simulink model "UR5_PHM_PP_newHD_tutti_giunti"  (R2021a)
settings: Solver=ode14x  StartTime=0.0  StopTime=Sim.time  FixedStep=Sim.dt  MaxStep=Sim.dt  RelTol=1e-3  EnableMultiTasking=on
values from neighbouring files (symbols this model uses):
  alpha_n = 0.98*pi/180    (= 0.0171042266695)    [parameters.m]
  alpha_t = 30*pi/180    (= 0.523598775598)    [parameters.m]
  alpha_TTS = 0    [parameters.m]
  alpha_Tw_L = -6.9e-4    (= -0.00069)    [parameters.m]
  alpha_Tw_R = 3.9e-3    (= 0.0039)    [parameters.m]
  Beta_TTS = 0    [parameters.m]
  c1 = 1e-2    (= 0.01)    [parameters.m]
  c2 = 1e-2    (= 0.01)    [parameters.m]
  c3 = 1e-2    (= 0.01)    [parameters.m]
  c4 = 1e-2    (= 0.01)    [parameters.m]
  c5 = 1e-2    (= 0.01)    [parameters.m]
  c6 = 1e-2    (= 0.01)    [parameters.m]
  Cb1 = 1.8e3    (= 1800)    [parameters.m]
  Cb2 = 1.8e3    (= 1800)    [parameters.m]
  Cb3 = 1.8e3    (= 1800)    [parameters.m]
  Cb4 = 1.8e3    (= 1800)    [parameters.m]
  Cb5 = 1.8e3    (= 1800)    [parameters.m]
  Cb6 = 1.8e3    (= 1800)    [parameters.m]
  Cth_housing = 153.90    (= 153.9)    [parameters.m]
  Cth_w = 74.20    (= 74.2)    [parameters.m]
  dt_PP = 0.05    [parameters.m]
  Fric1 = [fc_1/2 1e1 fc_1 fv_1]    [parameters.m]
  Fric2 = [fc_2/2 1e1 fc_2 fv_2]    [parameters.m]
  Fric3 = [fc_3/2 1e1 fc_3 fv_3]    [parameters.m]
  Fric4 = [fc_4/2 1e1 fc_4 fv_4]    [parameters.m]
  Fric5 = [fc_5/2 1e1 fc_5 fv_5]    [parameters.m]
  Fric6 = [fc_6/2 1e1 fc_6 fv_6]    [parameters.m]
  Hth_housing = 0.30    (= 0.3)    [parameters.m]
  Hth_w = 1.14    [parameters.m]
  I_actual = I_actual(1:10,:)    [trajcutting.m]
  J_CS1 = 7.12e-5    (= 7.12e-05)    [parameters.m]
  J_CS2 = 7.12e-5    (= 7.12e-05)    [parameters.m]
  J_CS3 = 7.12e-5    (= 7.12e-05)    [parameters.m]
  J_CS4 = 6e-6    (= 6e-06)    [parameters.m]
  J_CS5 = 6e-6    (= 6e-06)    [parameters.m]
  J_CS6 = 6e-6    (= 6e-06)    [parameters.m]
  J_FS1 = 1.62e-7    (= 1.62e-07)    [parameters.m]
  J_FS2 = 1.62e-7    (= 1.62e-07)    [parameters.m]
  J_FS3 = 1.62e-7    (= 1.62e-07)    [parameters.m]
  J_FS4 = 4.97e-8    (= 4.97e-08)    [parameters.m]
  J_FS5 = 4.97e-8    (= 4.97e-08)    [parameters.m]
  J_FS6 = 4.97e-8    (= 4.97e-08)    [parameters.m]
  J_WG1 = 3.56e-5    (= 3.56e-05)    [parameters.m]
  J_WG2 = 3.56e-5    (= 3.56e-05)    [parameters.m]
  J_WG3 = 3.56e-5    (= 3.56e-05)    [parameters.m]
  J_WG4 = 3e-6    (= 3e-06)    [parameters.m]
  J_WG5 = 3e-6    (= 3e-06)    [parameters.m]
  J_WG6 = 3e-6    (= 3e-06)    [parameters.m]
  K_i = 1    [parameters.m]
  K_p = 1    [parameters.m]
  K_torsCS1 = 4.78e6    (= 4780000)    [parameters.m]
  K_torsCS2 = 4.78e6    (= 4780000)    [parameters.m]
  K_torsCS3 = 4.78e6    (= 4780000)    [parameters.m]
  K_torsCS4 = 1.06e6    (= 1060000)    [parameters.m]
  K_torsCS5 = 1.06e6    (= 1060000)    [parameters.m]
  K_torsCS6 = 1.06e6    (= 1060000)    [parameters.m]
  K_torsWG1 = 9.56e5    (= 956000)    [parameters.m]
  K_torsWG2 = 9.56e5    (= 956000)    [parameters.m]
  K_torsWG3 = 9.56e5    (= 956000)    [parameters.m]
  K_torsWG4 = 1.84e5    (= 184000)    [parameters.m]
  K_torsWG5 = 1.84e5    (= 184000)    [parameters.m]
  K_torsWG6 = 1.84e5    (= 184000)    [parameters.m]
  K_v = 1    [parameters.m]
  Kb1 = 0.51e8    (= 51000000)    [parameters.m]
  Kb2 = 0.51e8    (= 51000000)    [parameters.m]
  Kb3 = 0.51e8    (= 51000000)    [parameters.m]
  Kb4 = 1.98e7    (= 19800000)    [parameters.m]
  Kb5 = 1.98e7    (= 19800000)    [parameters.m]
  Kb6 = 1.98e7    (= 19800000)    [parameters.m]
  Km1 = 1.2e9    (= 1200000000)    [parameters.m]
  Km2 = 1.2e9    (= 1200000000)    [parameters.m]
  Km3 = 1.2e9    (= 1200000000)    [parameters.m]
  Km4 = 5.55e8    (= 555000000)    [parameters.m]
  Km5 = 5.55e8    (= 555000000)    [parameters.m]
  Km6 = 5.55e8    (= 555000000)    [parameters.m]
  Kt1 = 0.96e5    (= 96000)    [parameters.m]
  Kt2 = 0.96e5    (= 96000)    [parameters.m]
  Kt3 = 0.96e5    (= 96000)    [parameters.m]
  Kt4 = 1.15e4    (= 11500)    [parameters.m]
  Kt5 = 1.15e4    (= 11500)    [parameters.m]
  Kt6 = 1.15e4    (= 11500)    [parameters.m]
  L = Motor.L_2/2    [parameters.m]
  m2 = polyfit(Temp(:,2),pBn_UR5_f_Temp(:,2),1)    [parameters.m]
  mb2 = polyfit(Temp(:,8),pBn_UR5_f_Temp(:,8),1)    [parameters.m]
  pickTime = t_pick(traj)    [parameters.m]
  placeTime = t_place(traj)    [parameters.m]
  q0 = q_target(1,:)    [testlaw_PP.m]
  q_CS01 = x(6)    [parameters.m]
  q_CS02 = x(6)    [parameters.m]
  q_CS03 = x(6)    [parameters.m]
  q_CS04 = x(6)    [parameters.m]
  q_CS05 = x(6)    [parameters.m]
  q_CS06 = x(6)    [parameters.m]
  q_WG01 = x(1)    [parameters.m]
  q_WG02 = x(1)    [parameters.m]
  q_WG03 = x(1)    [parameters.m]
  q_WG04 = x(1)    [parameters.m]
  q_WG05 = x(1)    [parameters.m]
  q_WG06 = x(1)    [parameters.m]
  quant_i = [Motor.imax1 Motor.imax2      Motor.imax3 Motor.imax4 Motor.imax5 Motor.imax6]/2^16    [parameters.m]
  R = Motor.R_2/2    [parameters.m]
  rg1 = 0.028    [parameters.m]
  rg2 = 0.028    [parameters.m]
  rg3 = 0.028    [parameters.m]
  rg4 = 0.0155    [parameters.m]
  rg5 = 0.0155    [parameters.m]
  rg6 = 0.0155    [parameters.m]
  sigma_p = 444.29    [parameters.m]
  sigma_v = 2*pi*1000    (= 6283.18530718)    [parameters.m]
  stiff_red = 1    [parameters.m]
  T_0 = Sim.temp    [parameters.m]
  T_switch = 1e-4    (= 0.0001)    [parameters.m]
  tau_i = 1/(fc_i*2*pi)    (= 7.95774715459e-05)    [parameters.m]
  U_s = 48    [parameters.m]
  var_i = 1e-1*[.0167 .0184 .0144 .0016      .0011 .0007]    [parameters.m]
  var_p = 1e-6*[.0943 .3877      .3478 .5436 .3400 .2081]    [parameters.m]
  var_v = 1e-4*[.0738 .1452      .1564 .4623 .1824 .0917]    [parameters.m]
  Wf_TTS_0 = 0    [parameters.m]
  Wf_TTS_ONOFF = 0    [parameters.m]
  x2_01 = x(3)    [parameters.m]
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undefined symbols (not defined in the file or in its folder): deg, Driver1, Driver2, Driver3, Driver4, Driver5, Driver6, elseif, geom, Ground, J1, J2, J3, J4, J5, J6, kg, L1, L2, L3, L4, L5, L6, LINK0, LINK1, LINK2, LINK3, LINK4, LINK5, LINK6, m, Motor, N, payload, ROBOTIQ_FT, s, Sim, Tool, X, Y, Z
libraries: sm_lib x35, nesl_utility x30, simulink x23, simulink_extras x11, spsTriangleGeneratorLib x6
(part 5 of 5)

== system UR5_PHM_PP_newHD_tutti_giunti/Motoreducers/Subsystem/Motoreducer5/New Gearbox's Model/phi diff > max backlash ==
  In2 : Inport
  In3 : Inport  Port=2
  Action Port : ActionPort  PropagateVarSize=During execution  ActionPortLabel=elseif(u2>u3)
  Add1 : Sum  Inputs=+|-
  Add2 : Sum  Inputs=+|+
  Add4 : Sum  Inputs=+|+
  Compare To Zero : simulink/Logic and Bit Operations/Compare To Zero  relop=<=  OutDataTypeStr=uint8
  Constant : Constant  Value=0
  Constant3 : Constant  Value=J5.clearance
  Cs_shaft [Nm/(rad/s)] : Gain  Gain=J5.C
  Ks_shaft [Nm/rad] : Gain  Gain=J5.K
  MinMax : MinMax  Inputs=2
  Switch : Switch  Criteria=u2 > Threshold
  Out1 : Outport  VectorParamsAs1DForOutWhenUnconnected=off
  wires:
  Switch/1 -> Out1/1
  Add2/1 -> Switch/3
  MinMax/1 -> Add2/2
  Add4/1 -> Compare To Zero/1
  Constant/1 -> Switch/1
  Compare To Zero/1 -> Switch/2
  Add1/1 -> Ks_shaft [Nm/rad]/1
  Constant3/1 -> Add1/2
  In2/1 -> Add1/1
  In3/1 -> Cs_shaft [Nm/(rad/s)]/1
  Cs_shaft [Nm/(rad/s)]/1 -> MinMax/2, Add4/2
  Ks_shaft [Nm/rad]/1 -> Add2/1, MinMax/1, Add4/1

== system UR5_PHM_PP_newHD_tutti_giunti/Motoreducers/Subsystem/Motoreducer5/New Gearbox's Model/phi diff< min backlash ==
  In2 : Inport
  In3 : Inport  Port=2
  Action Port : ActionPort  PropagateVarSize=During execution  ActionPortLabel=elseif( u2<u4)
  Add1 : Sum  Inputs=+|-
  Add2 : Sum  Inputs=+|+
  Add4 : Sum  Inputs=+|+
  Compare To Zero : simulink/Logic and Bit Operations/Compare To Zero  relop=>=  OutDataTypeStr=uint8
  Constant : Constant  Value=0
  Constant1 : Constant  Value=0
  Cs_shaft [Nm/(rad/s)] : Gain  Gain=J5.C
  Ks_shaft [Nm/rad] : Gain  Gain=J5.K
  MinMax : MinMax  Function=max  Inputs=2
  Switch : Switch  Criteria=u2 > Threshold
  Out1 : Outport  VectorParamsAs1DForOutWhenUnconnected=off
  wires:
  Switch/1 -> Out1/1
  Add2/1 -> Switch/3
  MinMax/1 -> Add2/2
  Add4/1 -> Compare To Zero/1
  Constant/1 -> Switch/1
  Compare To Zero/1 -> Switch/2
  Add1/1 -> Ks_shaft [Nm/rad]/1
  Constant1/1 -> Add1/2
  In2/1 -> Add1/1
  In3/1 -> Cs_shaft [Nm/(rad/s)]/1
  Cs_shaft [Nm/(rad/s)]/1 -> MinMax/2, Add4/2
  Ks_shaft [Nm/rad]/1 -> Add2/1, MinMax/1, Add4/1

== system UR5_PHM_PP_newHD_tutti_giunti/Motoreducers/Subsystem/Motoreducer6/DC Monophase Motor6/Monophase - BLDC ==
  Vset : Inport
  qdm : Inport  Port=2
  Phase A : Subsystem
  Torque constant [Nm/A] : Gain  Gain=Motor.kc_6
  T : Outport  VectorParamsAs1DForOutWhenUnconnected=off
  i : Outport  Port=2  VectorParamsAs1DForOutWhenUnconnected=off
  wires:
  Vset/1 -> Phase A/1(Vset)
  Torque constant [Nm/A]/1 -> T/1
  Phase A/1(i) -> Torque constant [Nm/A]/1, i/1
  qdm/1 -> Phase A/2(qdm)

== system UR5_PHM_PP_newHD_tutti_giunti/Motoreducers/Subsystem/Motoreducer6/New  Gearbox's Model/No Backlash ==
  qm : Inport
  q : Inport  Port=2
  qdm : Inport  Port=3
  qd : Inport  Port=4
  Action Port : ActionPort  PropagateVarSize=During execution  ActionPortLabel=if(u1<=1e-10)
  Circular spline : Subsystem
  Flexspline (rad) : Subsystem
  Flexspline (tang) : Subsystem
  Wave Generator : Subsystem
  Ccs->giunto : Outport
  Cwg->rotore : Outport  Port=2
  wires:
  Flexspline (tang)/1(y1) -> Flexspline (rad)/4(y1), Circular spline/1(y1)
  Flexspline (rad)/2(x2) -> Circular spline/3(x2), Flexspline (tang)/2(x2)
  q/1 -> Circular spline/4(q)
  qd/1 -> Circular spline/5(qd)
  Circular spline/1(C1) -> Ccs->giunto/1
  Circular spline/2(q_CS) -> Flexspline (rad)/3(q_CS)
  qm/1 -> Wave Generator/1(qm)
  qdm/1 -> Wave Generator/2(qdm)
  Flexspline (rad)/3(C_WG->FS) -> Wave Generator/3(C_FS->WG)
  Wave Generator/1(Cwg->rotore) -> Cwg->rotore/1
  Wave Generator/2(qm_WG) -> Flexspline (rad)/1(qm_WG)
  Wave Generator/3(qdm_WG) -> Flexspline (rad)/2(qdm_WG)
  Flexspline (rad)/1(y2) -> Circular spline/2(y2), Flexspline (tang)/1(y2)

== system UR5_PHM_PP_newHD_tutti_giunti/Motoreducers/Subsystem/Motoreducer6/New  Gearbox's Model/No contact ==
  In2 : Inport
  In3 : Inport  Port=2
  Action Port : ActionPort  PropagateVarSize=During execution  ActionPortLabel=else
  1/(2-1/eta_dir) : Gain  Gain=0
  Add4 : Sum  Inputs=+|+
  Out3 : Outport  VectorParamsAs1DForOutWhenUnconnected=off
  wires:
  Add4/1 -> 1/(2-1/eta_dir)/1
  In3/1 -> Add4/2
  In2/1 -> Add4/1
  1/(2-1/eta_dir)/1 -> Out3/1

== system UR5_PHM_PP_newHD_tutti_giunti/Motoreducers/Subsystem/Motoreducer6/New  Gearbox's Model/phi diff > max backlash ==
  In2 : Inport
  In3 : Inport  Port=2
  Action Port : ActionPort  PropagateVarSize=During execution  ActionPortLabel=elseif(u2>u3)
  Add1 : Sum  Inputs=+|-
  Add2 : Sum  Inputs=+|+
  Add4 : Sum  Inputs=+|+
  Compare To Zero : simulink/Logic and Bit Operations/Compare To Zero  relop=<=  OutDataTypeStr=uint8
  Constant : Constant  Value=0
  Constant3 : Constant  Value=J6.clearance
  Cs_shaft [Nm/(rad/s)] : Gain  Gain=J6.C
  Ks_shaft [Nm/rad] : Gain  Gain=J6.K
  MinMax : MinMax  Inputs=2
  Switch : Switch  Criteria=u2 > Threshold
  Out1 : Outport  VectorParamsAs1DForOutWhenUnconnected=off
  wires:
  Switch/1 -> Out1/1
  Add2/1 -> Switch/3
  MinMax/1 -> Add2/2
  Add4/1 -> Compare To Zero/1
  Constant/1 -> Switch/1
  Compare To Zero/1 -> Switch/2
  Add1/1 -> Ks_shaft [Nm/rad]/1
  Constant3/1 -> Add1/2
  In2/1 -> Add1/1
  In3/1 -> Cs_shaft [Nm/(rad/s)]/1
  Cs_shaft [Nm/(rad/s)]/1 -> MinMax/2, Add4/2
  Ks_shaft [Nm/rad]/1 -> Add2/1, MinMax/1, Add4/1

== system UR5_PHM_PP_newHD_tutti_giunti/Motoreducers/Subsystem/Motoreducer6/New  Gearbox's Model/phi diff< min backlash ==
  In2 : Inport
  In3 : Inport  Port=2
  Action Port : ActionPort  PropagateVarSize=During execution  ActionPortLabel=elseif( u2<u4)
  Add1 : Sum  Inputs=+|-
  Add2 : Sum  Inputs=+|+
  Add4 : Sum  Inputs=+|+
  Compare To Zero : simulink/Logic and Bit Operations/Compare To Zero  relop=>=  OutDataTypeStr=uint8
  Constant : Constant  Value=0
  Constant1 : Constant  Value=0
  Cs_shaft [Nm/(rad/s)] : Gain  Gain=J6.C
  Ks_shaft [Nm/rad] : Gain  Gain=J6.K
  MinMax : MinMax  Function=max  Inputs=2
  Switch : Switch  Criteria=u2 > Threshold
  Out1 : Outport  VectorParamsAs1DForOutWhenUnconnected=off
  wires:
  Switch/1 -> Out1/1
  Add2/1 -> Switch/3
  MinMax/1 -> Add2/2
  Add4/1 -> Compare To Zero/1
  Constant/1 -> Switch/1
  Compare To Zero/1 -> Switch/2
  Add1/1 -> Ks_shaft [Nm/rad]/1
  Constant1/1 -> Add1/2
  In2/1 -> Add1/1
  In3/1 -> Cs_shaft [Nm/(rad/s)]/1
  Cs_shaft [Nm/(rad/s)]/1 -> MinMax/2, Add4/2
  Ks_shaft [Nm/rad]/1 -> Add2/1, MinMax/1, Add4/1

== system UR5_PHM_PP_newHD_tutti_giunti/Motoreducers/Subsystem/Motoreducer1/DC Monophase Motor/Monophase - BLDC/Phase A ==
  Vset : Inport
  qdm : Inport  Port=2
  Add : Sum  Inputs=-+
  Gain : Gain  Gain=Motor.kv_1
  Saturation : Saturate  UpperLimit=Motor.imax1  LowerLimit=-Motor.imax1
  Transfer Fcn : TransferFcn  Numerator=[1/Motor.R_123]  Denominator=[Motor.L_123/Motor.R_123 1]
  i : Outport  VectorParamsAs1DForOutWhenUnconnected=off
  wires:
  Gain/1 -> Add/1
  Transfer Fcn/1 -> Saturation/1
  qdm/1 -> Gain/1
  Add/1 -> Transfer Fcn/1
  Vset/1 -> Add/2
  Saturation/1 -> i/1

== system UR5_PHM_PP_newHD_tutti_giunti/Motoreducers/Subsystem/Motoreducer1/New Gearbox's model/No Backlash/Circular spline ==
  y2 : Inport
  x2 : Inport  Port=2
  y1 : Inport  Port=3
  q : Inport  Port=4
  qd : Inport  Port=5
  1/J_CS : Gain  Gain=1/J_CS1
  Add : Sum  Inputs=+--
  Add1 : Sum  Inputs=+-
  Add2 : Sum  Inputs=+-
  Add3 : Sum
  Add4 : Sum  Inputs=-+-
  Integrator : Integrator
  Integrator1 : Integrator  InitialCondition=q_CS01
  K_torsCS : Gain  Gain=K_torsCS1
  c : Gain  Gain=c1
  cos(alpha_t) : Gain  Gain=cos(alpha_t)
  cos(alpha_t)2 : Gain  Gain=cos(alpha_t)
  rg*Km*cos(alpha_t) : Gain  Gain=rg1*Km1*cos(alpha_t)
  sin(alpha_t) : Gain  Gain=sin(alpha_t)
  C1 : Outport
  q_CS : Outport  Port=2
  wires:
  cos(alpha_t)/1 -> Add4/3
  Add4/1 -> rg*Km*cos(alpha_t)/1
  x2/1 -> sin(alpha_t)/1
  y1/1 -> cos(alpha_t)/1
  sin(alpha_t)/1 -> Add4/2
  cos(alpha_t)2/1 -> Add4/1
  y2/1 -> cos(alpha_t)2/1
  Integrator/1 -> Add2/1, Integrator1/1
  Add3/1 -> C1/1
  1/J_CS/1 -> Integrator/1
  Add1/1 -> K_torsCS/1
  Add/1 -> 1/J_CS/1
  Integrator1/1 -> q_CS/1, Add1/1
  c/1 -> Add3/2, Add/3
  K_torsCS/1 -> Add3/1, Add/2
  Add2/1 -> c/1
  rg*Km*cos(alpha_t)/1 -> Add/1
  qd/1 -> Add2/2
  q/1 -> Add1/2

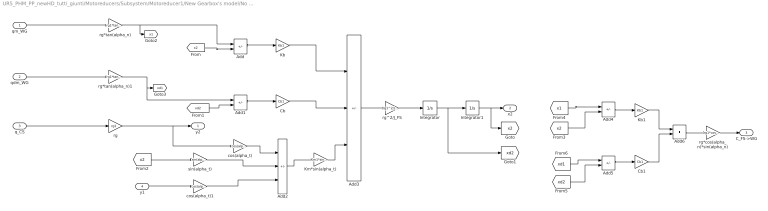
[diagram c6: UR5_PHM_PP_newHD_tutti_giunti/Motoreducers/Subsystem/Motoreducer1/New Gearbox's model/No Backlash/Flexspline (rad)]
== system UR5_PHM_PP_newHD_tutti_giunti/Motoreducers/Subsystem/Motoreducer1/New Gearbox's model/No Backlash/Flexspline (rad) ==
  qm_WG : Inport
  qdm_WG : Inport  Port=2
  q_CS : Inport  Port=3
  y1 : Inport  Port=4
  Add{,1,4..5} (4 alike) : Sum  Inputs=+-
  Add2 : Sum  Inputs=-+-
  Add3 : Sum  Inputs=++-
  Add6 : Sum
  Cb : Gain  Gain=Cb1
  Cb1 : Gain  Gain=Cb1
  Integrator : Integrator
  Integrator1 : Integrator  InitialCondition=x2_01
  Kb : Gain  Gain=Kb1
  Kb1 : Gain  Gain=Kb1
  Km*sin(alpha_t) : Gain  Gain=Km1*sin(alpha_t)
  cos(alpha_t) : Gain  Gain=cos(alpha_t)
  cos(alpha_t)1 : Gain  Gain=cos(alpha_t)
  rg : Gain  Gain=rg1
  rg*cos(alpha_n)*sin(alpha_n) : Gain  Gain=rg1*cos(alpha_n)*sin(alpha_n)
  rg*tan(alpha_n) : Gain  Gain=rg1*tan(alpha_n)
  rg*tan(alpha_n)1 : Gain  Gain=rg1*tan(alpha_n)
  rg^2/J_FS : Gain  Gain=rg1^2/J_FS1
  sin(alpha_t) : Gain  Gain=sin(alpha_t)
  y2 : Outport
  x2 : Outport  Port=2
  C_FS->WG : Outport  Port=3
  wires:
  Cb1/1 -> Add6/2
  Kb1/1 -> Add6/1
  sin(alpha_t)/1 -> Add2/2
  Add4/1 -> Kb1/1
  cos(alpha_t)1/1 -> Add2/3
  Add2/1 -> Km*sin(alpha_t)/1
  y1/1 -> cos(alpha_t)1/1
  Cb/1 -> Add3/2
  qdm_WG/1 -> rg*tan(alpha_n)1/1
  q_CS/1 -> rg/1
  Kb/1 -> Add3/1
  Km*sin(alpha_t)/1 -> Add3/3
  Add1/1 -> Cb/1
  rg/1 -> cos(alpha_t)/1, y2/1
  Integrator1/1 -> [x2], x2/1
  Add3/1 -> rg^2/J_FS/1
  rg^2/J_FS/1 -> Integrator/1
  cos(alpha_t)/1 -> Add2/1
  Add/1 -> Kb/1
  Integrator/1 -> [xd2], Integrator1/1
  Add5/1 -> Cb1/1
  [x2] -> sin(alpha_t)/1
  rg*tan(alpha_n)1/1 -> [xd1], Add1/1
  Add6/1 -> rg*cos(alpha_n)*sin(alpha_n)/1
  rg*cos(alpha_n)*sin(alpha_n)/1 -> C_FS->WG/1
  qm_WG/1 -> rg*tan(alpha_n)/1
  [xd2] -> Add1/2
  [x2] -> Add/2
  rg*tan(alpha_n)/1 -> [x1], Add/1
  [x2] -> Add4/2
  [x1] -> Add4/1
  [xd2] -> Add5/2
  [xd1] -> Add5/1

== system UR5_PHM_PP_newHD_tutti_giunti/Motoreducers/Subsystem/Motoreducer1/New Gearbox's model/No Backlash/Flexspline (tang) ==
  y2 : Inport
  x2 : Inport  Port=2
  Add : Sum  Inputs=+-
  Add4 : Sum  Inputs=-+-
  Integrator : Integrator
  Integrator1 : Integrator  InitialCondition=y1_01
  Km*cos(alpha_t) : Gain  Gain=Km1*cos(alpha_t)
  Kt/rg^2 : Gain  Gain=Kt1/rg1^2
  cos(alpha_t) : Gain  Gain=cos(alpha_t)
  cos(alpha_t)2 : Gain  Gain=cos(alpha_t)
  rg^2/J_FS : Gain  Gain=rg1^2/J_FS1
  sin(alpha_t) : Gain  Gain=sin(alpha_t)
  y1 : Outport
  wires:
  Integrator/1 -> Integrator1/1
  y2/1 -> cos(alpha_t)2/1
  Integrator1/1 -> cos(alpha_t)/1, Kt/rg^2/1, y1/1
  Add4/1 -> Km*cos(alpha_t)/1
  Kt/rg^2/1 -> Add/2
  rg^2/J_FS/1 -> Integrator/1
  Add/1 -> rg^2/J_FS/1
  x2/1 -> sin(alpha_t)/1
  Km*cos(alpha_t)/1 -> Add/1
  sin(alpha_t)/1 -> Add4/2
  cos(alpha_t)2/1 -> Add4/1
  cos(alpha_t)/1 -> Add4/3

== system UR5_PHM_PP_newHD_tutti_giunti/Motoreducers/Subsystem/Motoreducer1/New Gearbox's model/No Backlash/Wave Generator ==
  qm : Inport
  qdm : Inport  Port=2
  C_FS->WG : Inport  Port=3
  1/J_WG : Gain  Gain=1/J_WG1
  Add : Sum  Inputs=+-
  Add1 : Sum  Inputs=+-
  Add2 : Sum
  Add4 : Sum  Inputs=+-
  Integrator1 : Integrator
  Integrator2 : Integrator  InitialCondition=q_WG01
  K_torsWG : Gain  Gain=K_torsWG1
  c : Gain  Gain=c1
  Cwg->rotore : Outport
  qm_WG : Outport  Port=2
  qdm_WG : Outport  Port=3
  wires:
  Integrator1/1 -> qdm_WG/1, Add1/2, Integrator2/1
  Add1/1 -> c/1
  Integrator2/1 -> qm_WG/1, Add/2
  Add2/1 -> Cwg->rotore/1, Add4/1
  1/J_WG/1 -> Integrator1/1
  c/1 -> Add2/2
  Add4/1 -> 1/J_WG/1
  Add/1 -> K_torsWG/1
  K_torsWG/1 -> Add2/1
  C_FS->WG/1 -> Add4/2
  qm/1 -> Add/1
  qdm/1 -> Add1/1

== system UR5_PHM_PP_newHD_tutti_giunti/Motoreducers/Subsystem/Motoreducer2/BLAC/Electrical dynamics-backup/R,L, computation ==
  Tw [°C] : Inport
  Add : Sum  Inputs=-+
  Constant : Constant
  Fcn : Fcn  Expr=(u(1)-Sim.temp)*alpha_Tw_R*R+R
  Fcn1 : Fcn  Expr=(u(1)-Sim.temp)*alpha_Tw_L*L+L
  Multiply : Product
  Multiply1 : Product
  Mux : Mux  Inputs=[1;1;1]
  Mux1 : Mux  Inputs=[1;1;1]
  Sqrt : Sqrt
  TTS_phase a : Subsystem
  L[a,b,c] : Outport  VectorParamsAs1DForOutWhenUnconnected=off
  R[a,b,c] : Outport  Port=2  VectorParamsAs1DForOutWhenUnconnected=off
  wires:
  Tw [°C]/1 -> TTS_phase a/1(Tw [°C]), Fcn/1, Fcn1/1
  TTS_phase a/1(Wf) -> Add/1
  Constant/1 -> Add/2
  Fcn/1 -> Mux/3, Mux/2, Multiply/1
  Mux/1 -> R[a,b,c]/1
  Add/1 -> Sqrt/1, Multiply/2
  Multiply/1 -> Mux/1
  Fcn1/1 -> Multiply1/2, Mux1/3, Mux1/2
  Sqrt/1 -> Multiply1/1
  Multiply1/1 -> Mux1/1
  Mux1/1 -> L[a,b,c]/1

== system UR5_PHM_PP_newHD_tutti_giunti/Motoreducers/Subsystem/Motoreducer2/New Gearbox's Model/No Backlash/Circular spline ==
  y1 : Inport
  y2 : Inport  Port=2
  x2 : Inport  Port=3
  q : Inport  Port=4
  qd : Inport  Port=5
  1/J_CS : Gain  Gain=1/J_CS2
  Add : Sum  Inputs=+--
  Add1 : Sum  Inputs=+-
  Add2 : Sum  Inputs=+-
  Add3 : Sum
  Add4 : Sum  Inputs=-+-
  Integrator : Integrator
  Integrator1 : Integrator  InitialCondition=q_CS02
  K_torsCS : Gain  Gain=K_torsCS2
  c : Gain  Gain=c2
  cos(alpha_t) : Gain  Gain=cos(alpha_t)
  cos(alpha_t)2 : Gain  Gain=cos(alpha_t)
  rg*Km*cos(alpha_t) : Gain  Gain=rg2*Km2*cos(alpha_t)
  sin(alpha_t) : Gain  Gain=sin(alpha_t)
  C1 : Outport
  q_CS : Outport  Port=2
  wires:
  cos(alpha_t)/1 -> Add4/3
  Add4/1 -> rg*Km*cos(alpha_t)/1
  x2/1 -> sin(alpha_t)/1
  y1/1 -> cos(alpha_t)/1
  sin(alpha_t)/1 -> Add4/2
  cos(alpha_t)2/1 -> Add4/1
  y2/1 -> cos(alpha_t)2/1
  K_torsCS/1 -> Add3/1, Add/2
  1/J_CS/1 -> Integrator/1
  Add/1 -> 1/J_CS/1
  Add3/1 -> C1/1
  Integrator/1 -> Add2/1, Integrator1/1
  Integrator1/1 -> q_CS/1, Add1/1
  qd/1 -> Add2/2
  Add2/1 -> c/1
  Add1/1 -> K_torsCS/1
  q/1 -> Add1/2
  c/1 -> Add3/2, Add/3
  rg*Km*cos(alpha_t)/1 -> Add/1

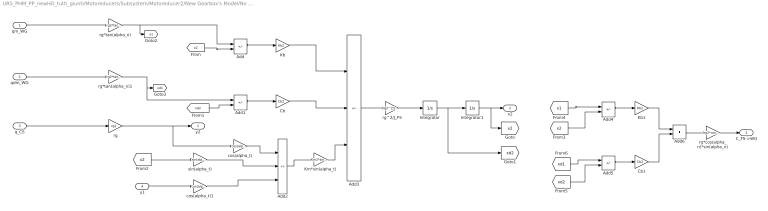
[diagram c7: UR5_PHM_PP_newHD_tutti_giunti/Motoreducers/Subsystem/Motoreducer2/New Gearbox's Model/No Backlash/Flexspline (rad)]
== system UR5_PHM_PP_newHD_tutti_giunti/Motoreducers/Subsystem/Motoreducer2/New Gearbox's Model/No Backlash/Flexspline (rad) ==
  qm_WG : Inport
  qdm_WG : Inport  Port=2
  q_CS : Inport  Port=3
  y1 : Inport  Port=4
  Add{,1,4..5} (4 alike) : Sum  Inputs=+-
  Add2 : Sum  Inputs=-+-
  Add3 : Sum  Inputs=++-
  Add6 : Sum
  Cb : Gain  Gain=Cb2
  Cb1 : Gain  Gain=Cb2
  Integrator : Integrator
  Integrator1 : Integrator  InitialCondition=x2_02
  Kb : Gain  Gain=Kb2
  Kb1 : Gain  Gain=Kb2
  Km*sin(alpha_t) : Gain  Gain=Km2*sin(alpha_t)
  cos(alpha_t) : Gain  Gain=cos(alpha_t)
  cos(alpha_t)1 : Gain  Gain=cos(alpha_t)
  rg : Gain  Gain=rg2
  rg*cos(alpha_n)*sin(alpha_n) : Gain  Gain=rg2*cos(alpha_n)*sin(alpha_n)
  rg*tan(alpha_n) : Gain  Gain=rg2*tan(alpha_n)
  rg*tan(alpha_n)1 : Gain  Gain=rg2*tan(alpha_n)
  rg^2/J_FS : Gain  Gain=rg2^2/J_FS2
  sin(alpha_t) : Gain  Gain=sin(alpha_t)
  y2 : Outport
  x2 : Outport  Port=2
  C_FS->WG : Outport  Port=3
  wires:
  Cb1/1 -> Add6/2
  Kb1/1 -> Add6/1
  sin(alpha_t)/1 -> Add2/2
  Add4/1 -> Kb1/1
  cos(alpha_t)1/1 -> Add2/3
  Add2/1 -> Km*sin(alpha_t)/1
  y1/1 -> cos(alpha_t)1/1
  Cb/1 -> Add3/2
  qdm_WG/1 -> rg*tan(alpha_n)1/1
  q_CS/1 -> rg/1
  Kb/1 -> Add3/1
  Km*sin(alpha_t)/1 -> Add3/3
  Add1/1 -> Cb/1
  rg/1 -> cos(alpha_t)/1, y2/1
  Integrator1/1 -> [x2], x2/1
  Add3/1 -> rg^2/J_FS/1
  rg^2/J_FS/1 -> Integrator/1
  cos(alpha_t)/1 -> Add2/1
  Add/1 -> Kb/1
  Integrator/1 -> [xd2], Integrator1/1
  Add5/1 -> Cb1/1
  [x2] -> sin(alpha_t)/1
  rg*tan(alpha_n)1/1 -> [xd1], Add1/1
  Add6/1 -> rg*cos(alpha_n)*sin(alpha_n)/1
  rg*cos(alpha_n)*sin(alpha_n)/1 -> C_FS->WG/1
  qm_WG/1 -> rg*tan(alpha_n)/1
  [xd2] -> Add1/2
  [x2] -> Add/2
  rg*tan(alpha_n)/1 -> [x1], Add/1
  [x2] -> Add4/2
  [x1] -> Add4/1
  [xd2] -> Add5/2
  [xd1] -> Add5/1

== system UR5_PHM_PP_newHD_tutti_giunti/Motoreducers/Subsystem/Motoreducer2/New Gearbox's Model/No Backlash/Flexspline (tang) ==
  y2 : Inport
  x2 : Inport  Port=2
  Add : Sum  Inputs=+-
  Add4 : Sum  Inputs=-+-
  Integrator : Integrator
  Integrator1 : Integrator  InitialCondition=y1_02
  Km*cos(alpha_t) : Gain  Gain=Km2*cos(alpha_t)
  Kt/rg^2 : Gain  Gain=Kt2/rg2^2
  cos(alpha_t) : Gain  Gain=cos(alpha_t)
  cos(alpha_t)2 : Gain  Gain=cos(alpha_t)
  rg^2/J_FS : Gain  Gain=rg2^2/J_FS2
  sin(alpha_t) : Gain  Gain=sin(alpha_t)
  y1 : Outport
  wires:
  Integrator/1 -> Integrator1/1
  y2/1 -> cos(alpha_t)2/1
  Integrator1/1 -> cos(alpha_t)/1, Kt/rg^2/1, y1/1
  Add4/1 -> Km*cos(alpha_t)/1
  Kt/rg^2/1 -> Add/2
  rg^2/J_FS/1 -> Integrator/1
  Add/1 -> rg^2/J_FS/1
  x2/1 -> sin(alpha_t)/1
  Km*cos(alpha_t)/1 -> Add/1
  sin(alpha_t)/1 -> Add4/2
  cos(alpha_t)2/1 -> Add4/1
  cos(alpha_t)/1 -> Add4/3

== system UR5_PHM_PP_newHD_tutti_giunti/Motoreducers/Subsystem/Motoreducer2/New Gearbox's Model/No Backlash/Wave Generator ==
  qm : Inport
  qdm : Inport  Port=2
  C_FS->WG : Inport  Port=3
  1/J_WG : Gain  Gain=1/J_WG2
  Add : Sum  Inputs=+-
  Add1 : Sum  Inputs=+-
  Add2 : Sum
  Add4 : Sum  Inputs=+-
  Integrator1 : Integrator
  Integrator2 : Integrator  InitialCondition=q_WG02
  K_torsWG : Gain  Gain=K_torsWG2
  c : Gain  Gain=c2
  C_wg->rotore : Outport
  qm_WG : Outport  Port=2
  qdm_WG : Outport  Port=3
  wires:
  c/1 -> Add2/2
  1/J_WG/1 -> Integrator1/1
  K_torsWG/1 -> Add2/1
  Integrator1/1 -> qdm_WG/1, Add1/2, Integrator2/1
  Integrator2/1 -> qm_WG/1, Add/2
  Add2/1 -> C_wg->rotore/1, Add4/1
  Add1/1 -> c/1
  qdm/1 -> Add1/1
  Add4/1 -> 1/J_WG/1
  Add/1 -> K_torsWG/1
  C_FS->WG/1 -> Add4/2
  qm/1 -> Add/1

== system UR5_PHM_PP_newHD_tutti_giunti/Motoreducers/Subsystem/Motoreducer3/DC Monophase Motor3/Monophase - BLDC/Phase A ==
  Vset : Inport
  qdm : Inport  Port=2
  Add : Sum  Inputs=-+
  Gain : Gain  Gain=Motor.kv_3
  Saturation : Saturate  UpperLimit=Motor.imax3  LowerLimit=-Motor.imax3
  Transfer Fcn : TransferFcn  Numerator=[1/Motor.R_123]  Denominator=[Motor.L_123/Motor.R_123 1]
  i : Outport  VectorParamsAs1DForOutWhenUnconnected=off
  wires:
  Gain/1 -> Add/1
  Transfer Fcn/1 -> Saturation/1
  qdm/1 -> Gain/1
  Add/1 -> Transfer Fcn/1
  Vset/1 -> Add/2
  Saturation/1 -> i/1

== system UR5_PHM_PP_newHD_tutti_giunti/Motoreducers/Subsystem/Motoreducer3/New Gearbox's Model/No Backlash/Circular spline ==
  y1 : Inport
  y2 : Inport  Port=2
  x2 : Inport  Port=3
  q : Inport  Port=4
  qd : Inport  Port=5
  1/J_CS : Gain  Gain=1/J_CS3
  Add : Sum  Inputs=+--
  Add1 : Sum  Inputs=+-
  Add2 : Sum  Inputs=+-
  Add3 : Sum
  Add4 : Sum  Inputs=-+-
  Integrator : Integrator
  Integrator1 : Integrator  InitialCondition=q_CS03
  K_torsCS : Gain  Gain=K_torsCS3
  c : Gain  Gain=c3
  cos(alpha_t) : Gain  Gain=cos(alpha_t)
  cos(alpha_t)2 : Gain  Gain=cos(alpha_t)
  rg*Km*cos(alpha_t) : Gain  Gain=rg3*Km3*cos(alpha_t)
  sin(alpha_t) : Gain  Gain=sin(alpha_t)
  C1 : Outport
  q_CS : Outport  Port=2
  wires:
  cos(alpha_t)/1 -> Add4/3
  Add4/1 -> rg*Km*cos(alpha_t)/1
  x2/1 -> sin(alpha_t)/1
  y1/1 -> cos(alpha_t)/1
  sin(alpha_t)/1 -> Add4/2
  cos(alpha_t)2/1 -> Add4/1
  y2/1 -> cos(alpha_t)2/1
  c/1 -> Add3/2, Add/3
  Add1/1 -> K_torsCS/1
  Add2/1 -> c/1
  rg*Km*cos(alpha_t)/1 -> Add/1
  Add3/1 -> C1/1
  Integrator/1 -> Add2/1, Integrator1/1
  1/J_CS/1 -> Integrator/1
  Add/1 -> 1/J_CS/1
  K_torsCS/1 -> Add3/1, Add/2
  Integrator1/1 -> q_CS/1, Add1/1
  qd/1 -> Add2/2
  q/1 -> Add1/2

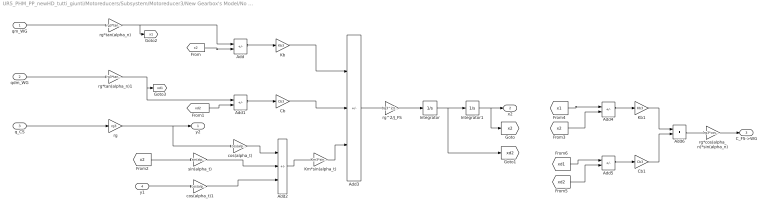
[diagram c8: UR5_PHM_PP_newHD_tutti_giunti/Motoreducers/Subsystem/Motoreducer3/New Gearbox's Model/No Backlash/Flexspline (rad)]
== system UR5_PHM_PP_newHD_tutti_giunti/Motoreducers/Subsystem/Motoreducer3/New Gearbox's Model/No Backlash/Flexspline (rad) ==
  qm_WG : Inport
  qdm_WG : Inport  Port=2
  q_CS : Inport  Port=3
  y1 : Inport  Port=4
  Add{,1,4..5} (4 alike) : Sum  Inputs=+-
  Add2 : Sum  Inputs=-+-
  Add3 : Sum  Inputs=++-
  Add6 : Sum
  Cb : Gain  Gain=Cb3
  Cb1 : Gain  Gain=Cb3
  Integrator : Integrator
  Integrator1 : Integrator  InitialCondition=x2_03
  Kb : Gain  Gain=Kb3
  Kb1 : Gain  Gain=Kb3
  Km*sin(alpha_t) : Gain  Gain=Km3*sin(alpha_t)
  cos(alpha_t) : Gain  Gain=cos(alpha_t)
  cos(alpha_t)1 : Gain  Gain=cos(alpha_t)
  rg : Gain  Gain=rg3
  rg*cos(alpha_n)*sin(alpha_n) : Gain  Gain=rg3*cos(alpha_n)*sin(alpha_n)
  rg*tan(alpha_n) : Gain  Gain=rg3*tan(alpha_n)
  rg*tan(alpha_n)1 : Gain  Gain=rg3*tan(alpha_n)
  rg^2/J_FS : Gain  Gain=rg3^2/J_FS3
  sin(alpha_t) : Gain  Gain=sin(alpha_t)
  y2 : Outport
  x2 : Outport  Port=2
  C_FS->WG : Outport  Port=3
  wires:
  Cb1/1 -> Add6/2
  Kb1/1 -> Add6/1
  sin(alpha_t)/1 -> Add2/2
  Add4/1 -> Kb1/1
  cos(alpha_t)1/1 -> Add2/3
  Add2/1 -> Km*sin(alpha_t)/1
  y1/1 -> cos(alpha_t)1/1
  Cb/1 -> Add3/2
  qdm_WG/1 -> rg*tan(alpha_n)1/1
  q_CS/1 -> rg/1
  Kb/1 -> Add3/1
  Km*sin(alpha_t)/1 -> Add3/3
  Add1/1 -> Cb/1
  rg/1 -> cos(alpha_t)/1, y2/1
  Integrator1/1 -> [x2], x2/1
  Add3/1 -> rg^2/J_FS/1
  rg^2/J_FS/1 -> Integrator/1
  cos(alpha_t)/1 -> Add2/1
  Add/1 -> Kb/1
  Integrator/1 -> [xd2], Integrator1/1
  Add5/1 -> Cb1/1
  [x2] -> sin(alpha_t)/1
  rg*tan(alpha_n)1/1 -> [xd1], Add1/1
  Add6/1 -> rg*cos(alpha_n)*sin(alpha_n)/1
  rg*cos(alpha_n)*sin(alpha_n)/1 -> C_FS->WG/1
  qm_WG/1 -> rg*tan(alpha_n)/1
  [xd2] -> Add1/2
  [x2] -> Add/2
  rg*tan(alpha_n)/1 -> [x1], Add/1
  [x2] -> Add4/2
  [x1] -> Add4/1
  [xd2] -> Add5/2
  [xd1] -> Add5/1

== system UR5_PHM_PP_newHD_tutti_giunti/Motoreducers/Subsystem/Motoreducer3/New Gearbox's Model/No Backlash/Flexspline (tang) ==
  y2 : Inport
  x2 : Inport  Port=2
  Add : Sum  Inputs=+-
  Add4 : Sum  Inputs=-+-
  Integrator : Integrator
  Integrator1 : Integrator  InitialCondition=y1_03
  Km*cos(alpha_t) : Gain  Gain=Km3*cos(alpha_t)
  Kt/rg^2 : Gain  Gain=Kt3/rg3^2
  cos(alpha_t) : Gain  Gain=cos(alpha_t)
  cos(alpha_t)2 : Gain  Gain=cos(alpha_t)
  rg^2/J_FS : Gain  Gain=rg3^2/J_FS3
  sin(alpha_t) : Gain  Gain=sin(alpha_t)
  y1 : Outport
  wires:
  Integrator/1 -> Integrator1/1
  y2/1 -> cos(alpha_t)2/1
  Integrator1/1 -> cos(alpha_t)/1, Kt/rg^2/1, y1/1
  Add4/1 -> Km*cos(alpha_t)/1
  Kt/rg^2/1 -> Add/2
  rg^2/J_FS/1 -> Integrator/1
  Add/1 -> rg^2/J_FS/1
  x2/1 -> sin(alpha_t)/1
  Km*cos(alpha_t)/1 -> Add/1
  sin(alpha_t)/1 -> Add4/2
  cos(alpha_t)2/1 -> Add4/1
  cos(alpha_t)/1 -> Add4/3

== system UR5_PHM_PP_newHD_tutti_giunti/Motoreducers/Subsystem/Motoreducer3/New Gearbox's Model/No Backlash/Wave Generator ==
  qm : Inport
  qdm : Inport  Port=2
  C_FS->WG : Inport  Port=3
  1/J_WG : Gain  Gain=1/J_WG3
  Add : Sum  Inputs=+-
  Add1 : Sum  Inputs=+-
  Add2 : Sum
  Add4 : Sum  Inputs=+-
  Integrator1 : Integrator
  Integrator2 : Integrator  InitialCondition=q_WG03
  K_torsWG : Gain  Gain=K_torsWG3
  c : Gain  Gain=c3
  Cwg->rotore : Outport
  qm_WG : Outport  Port=2
  qdm_WG : Outport  Port=3
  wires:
  1/J_WG/1 -> Integrator1/1
  Add4/1 -> 1/J_WG/1
  Integrator1/1 -> qdm_WG/1, Add1/2, Integrator2/1
  K_torsWG/1 -> Add2/1
  c/1 -> Add2/2
  Add2/1 -> Cwg->rotore/1, Add4/1
  qdm/1 -> Add1/1
  Add1/1 -> c/1
  Integrator2/1 -> qm_WG/1, Add/2
  qm/1 -> Add/1
  Add/1 -> K_torsWG/1
  C_FS->WG/1 -> Add4/2

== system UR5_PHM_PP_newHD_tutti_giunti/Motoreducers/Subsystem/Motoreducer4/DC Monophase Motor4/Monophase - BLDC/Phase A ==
  Vset : Inport
  qdm : Inport  Port=2
  Add : Sum  Inputs=-+
  Gain : Gain  Gain=Motor.kv_4
  Saturation : Saturate  UpperLimit=Motor.imax4  LowerLimit=-Motor.imax4
  Transfer Fcn : TransferFcn  Numerator=[1/Motor.R_456]  Denominator=[Motor.L_456/Motor.R_456 1]
  i : Outport  VectorParamsAs1DForOutWhenUnconnected=off
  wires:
  Gain/1 -> Add/1
  Transfer Fcn/1 -> Saturation/1
  qdm/1 -> Gain/1
  Add/1 -> Transfer Fcn/1
  Vset/1 -> Add/2
  Saturation/1 -> i/1

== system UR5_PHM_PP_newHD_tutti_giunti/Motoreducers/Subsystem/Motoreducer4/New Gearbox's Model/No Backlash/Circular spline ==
  y1 : Inport
  y2 : Inport  Port=2
  x2 : Inport  Port=3
  q : Inport  Port=4
  qd : Inport  Port=5
  1/J_CS : Gain  Gain=1/J_CS4
  Add : Sum  Inputs=+--
  Add1 : Sum  Inputs=+-
  Add2 : Sum  Inputs=+-
  Add3 : Sum
  Add4 : Sum  Inputs=-+-
  Integrator : Integrator
  Integrator1 : Integrator  InitialCondition=q_CS04
  K_torsCS : Gain  Gain=K_torsCS4
  c : Gain  Gain=c4
  cos(alpha_t) : Gain  Gain=cos(alpha_t)
  cos(alpha_t)2 : Gain  Gain=cos(alpha_t)
  rg*Km*cos(alpha_t) : Gain  Gain=rg4*Km4*cos(alpha_t)
  sin(alpha_t) : Gain  Gain=sin(alpha_t)
  C1 : Outport
  q_CS : Outport  Port=2
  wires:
  cos(alpha_t)/1 -> Add4/3
  Add4/1 -> rg*Km*cos(alpha_t)/1
  x2/1 -> sin(alpha_t)/1
  y1/1 -> cos(alpha_t)/1
  sin(alpha_t)/1 -> Add4/2
  cos(alpha_t)2/1 -> Add4/1
  y2/1 -> cos(alpha_t)2/1
  Integrator1/1 -> q_CS/1, Add1/1
  K_torsCS/1 -> Add3/1, Add/2
  Integrator/1 -> Add2/1, Integrator1/1
  Add3/1 -> C1/1
  Add/1 -> 1/J_CS/1
  Add2/1 -> c/1
  c/1 -> Add3/2, Add/3
  1/J_CS/1 -> Integrator/1
  Add1/1 -> K_torsCS/1
  rg*Km*cos(alpha_t)/1 -> Add/1
  q/1 -> Add1/2
  qd/1 -> Add2/2

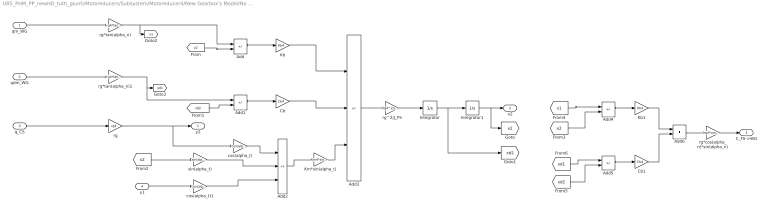
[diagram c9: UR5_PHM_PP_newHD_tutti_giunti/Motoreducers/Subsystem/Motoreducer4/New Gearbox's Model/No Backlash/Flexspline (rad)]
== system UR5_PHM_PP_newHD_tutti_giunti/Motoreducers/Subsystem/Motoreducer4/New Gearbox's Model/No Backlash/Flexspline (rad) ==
  qm_WG : Inport
  qdm_WG : Inport  Port=2
  q_CS : Inport  Port=3
  y1 : Inport  Port=4
  Add{,1,4..5} (4 alike) : Sum  Inputs=+-
  Add2 : Sum  Inputs=-+-
  Add3 : Sum  Inputs=++-
  Add6 : Sum
  Cb : Gain  Gain=Cb4
  Cb1 : Gain  Gain=Cb4
  Integrator : Integrator
  Integrator1 : Integrator  InitialCondition=x2_04
  Kb : Gain  Gain=Kb4
  Kb1 : Gain  Gain=Kb4
  Km*sin(alpha_t) : Gain  Gain=Km4*sin(alpha_t)
  cos(alpha_t) : Gain  Gain=cos(alpha_t)
  cos(alpha_t)1 : Gain  Gain=cos(alpha_t)
  rg : Gain  Gain=rg4
  rg*cos(alpha_n)*sin(alpha_n) : Gain  Gain=rg4*cos(alpha_n)*sin(alpha_n)
  rg*tan(alpha_n) : Gain  Gain=rg4*tan(alpha_n)
  rg*tan(alpha_n)1 : Gain  Gain=rg4*tan(alpha_n)
  rg^2/J_FS : Gain  Gain=rg4^2/J_FS4
  sin(alpha_t) : Gain  Gain=sin(alpha_t)
  y2 : Outport
  x2 : Outport  Port=2
  C_FS->WG : Outport  Port=3
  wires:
  Cb1/1 -> Add6/2
  Kb1/1 -> Add6/1
  sin(alpha_t)/1 -> Add2/2
  Add4/1 -> Kb1/1
  cos(alpha_t)1/1 -> Add2/3
  Add2/1 -> Km*sin(alpha_t)/1
  y1/1 -> cos(alpha_t)1/1
  Cb/1 -> Add3/2
  qdm_WG/1 -> rg*tan(alpha_n)1/1
  q_CS/1 -> rg/1
  Kb/1 -> Add3/1
  Km*sin(alpha_t)/1 -> Add3/3
  Add1/1 -> Cb/1
  rg/1 -> cos(alpha_t)/1, y2/1
  Integrator1/1 -> [x2], x2/1
  Add3/1 -> rg^2/J_FS/1
  rg^2/J_FS/1 -> Integrator/1
  cos(alpha_t)/1 -> Add2/1
  Add/1 -> Kb/1
  Integrator/1 -> [xd2], Integrator1/1
  Add5/1 -> Cb1/1
  [x2] -> sin(alpha_t)/1
  rg*tan(alpha_n)1/1 -> [xd1], Add1/1
  Add6/1 -> rg*cos(alpha_n)*sin(alpha_n)/1
  rg*cos(alpha_n)*sin(alpha_n)/1 -> C_FS->WG/1
  qm_WG/1 -> rg*tan(alpha_n)/1
  [xd2] -> Add1/2
  [x2] -> Add/2
  rg*tan(alpha_n)/1 -> [x1], Add/1
  [x2] -> Add4/2
  [x1] -> Add4/1
  [xd2] -> Add5/2
  [xd1] -> Add5/1

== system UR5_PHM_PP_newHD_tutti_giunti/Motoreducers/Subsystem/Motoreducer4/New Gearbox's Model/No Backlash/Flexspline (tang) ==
  y2 : Inport
  x2 : Inport  Port=2
  Add : Sum  Inputs=+-
  Add4 : Sum  Inputs=-+-
  Integrator : Integrator
  Integrator1 : Integrator  InitialCondition=y1_04
  Km*cos(alpha_t) : Gain  Gain=Km4*cos(alpha_t)
  Kt/rg^2 : Gain  Gain=Kt4/rg4^2
  cos(alpha_t) : Gain  Gain=cos(alpha_t)
  cos(alpha_t)2 : Gain  Gain=cos(alpha_t)
  rg^2/J_FS : Gain  Gain=rg4^2/J_FS4
  sin(alpha_t) : Gain  Gain=sin(alpha_t)
  y1 : Outport
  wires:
  Integrator/1 -> Integrator1/1
  y2/1 -> cos(alpha_t)2/1
  Add4/1 -> Km*cos(alpha_t)/1
  Kt/rg^2/1 -> Add/2
  rg^2/J_FS/1 -> Integrator/1
  Add/1 -> rg^2/J_FS/1
  x2/1 -> sin(alpha_t)/1
  Km*cos(alpha_t)/1 -> Add/1
  sin(alpha_t)/1 -> Add4/2
  cos(alpha_t)2/1 -> Add4/1
  cos(alpha_t)/1 -> Add4/3
  Integrator1/1 -> cos(alpha_t)/1, Kt/rg^2/1, y1/1

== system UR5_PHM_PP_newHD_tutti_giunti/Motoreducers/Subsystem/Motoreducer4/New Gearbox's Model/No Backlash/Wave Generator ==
  qm : Inport
  qdm : Inport  Port=2
  C_FS->WG : Inport  Port=3
  1/J_WG : Gain  Gain=1/J_WG4
  Add : Sum  Inputs=+-
  Add1 : Sum  Inputs=+-
  Add2 : Sum
  Add4 : Sum  Inputs=+-
  Integrator1 : Integrator
  Integrator2 : Integrator  InitialCondition=q_WG04
  K_torsWG : Gain  Gain=K_torsWG4
  c : Gain  Gain=c4
  qm_WG : Outport
  Cwg->rotore : Outport  Port=2
  qdm_WG : Outport  Port=3
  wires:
  Add1/1 -> c/1
  Add2/1 -> Cwg->rotore/1, Add4/1
  Add/1 -> K_torsWG/1
  1/J_WG/1 -> Integrator1/1
  K_torsWG/1 -> Add2/1
  c/1 -> Add2/2
  C_FS->WG/1 -> Add4/2
  Integrator1/1 -> qdm_WG/1, Add1/2, Integrator2/1
  Integrator2/1 -> qm_WG/1, Add/2
  Add4/1 -> 1/J_WG/1
  qdm/1 -> Add1/1
  qm/1 -> Add/1

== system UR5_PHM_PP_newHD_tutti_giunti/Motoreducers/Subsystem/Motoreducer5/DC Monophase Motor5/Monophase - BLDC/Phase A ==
  Vset : Inport
  qdm : Inport  Port=2
  Add : Sum  Inputs=-+
  Gain : Gain  Gain=Motor.kv_5
  Saturation : Saturate  UpperLimit=Motor.imax5  LowerLimit=-Motor.imax5
  Transfer Fcn : TransferFcn  Numerator=[1/Motor.R_456]  Denominator=[Motor.L_456/Motor.R_456 1]
  i : Outport  VectorParamsAs1DForOutWhenUnconnected=off
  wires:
  Gain/1 -> Add/1
  Transfer Fcn/1 -> Saturation/1
  qdm/1 -> Gain/1
  Add/1 -> Transfer Fcn/1
  Vset/1 -> Add/2
  Saturation/1 -> i/1

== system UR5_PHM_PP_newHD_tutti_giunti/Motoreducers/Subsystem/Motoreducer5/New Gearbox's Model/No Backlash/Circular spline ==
  y1 : Inport
  y2 : Inport  Port=2
  x2 : Inport  Port=3
  q : Inport  Port=4
  qd : Inport  Port=5
  1/J_CS : Gain  Gain=1/J_CS5
  Add : Sum  Inputs=+--
  Add1 : Sum  Inputs=+-
  Add2 : Sum  Inputs=+-
  Add3 : Sum
  Add4 : Sum  Inputs=-+-
  Integrator : Integrator
  Integrator1 : Integrator  InitialCondition=q_CS05
  K_torsCS : Gain  Gain=K_torsCS5
  c : Gain  Gain=c5
  cos(alpha_t) : Gain  Gain=cos(alpha_t)
  cos(alpha_t)2 : Gain  Gain=cos(alpha_t)
  rg*Km*cos(alpha_t) : Gain  Gain=rg5*Km5*cos(alpha_t)
  sin(alpha_t) : Gain  Gain=sin(alpha_t)
  C1 : Outport
  q_CS : Outport  Port=2
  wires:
  cos(alpha_t)/1 -> Add4/3
  Add4/1 -> rg*Km*cos(alpha_t)/1
  x2/1 -> sin(alpha_t)/1
  y1/1 -> cos(alpha_t)/1
  sin(alpha_t)/1 -> Add4/2
  cos(alpha_t)2/1 -> Add4/1
  y2/1 -> cos(alpha_t)2/1
  rg*Km*cos(alpha_t)/1 -> Add/1
  q/1 -> Add1/2
  Integrator1/1 -> q_CS/1, Add1/1
  K_torsCS/1 -> Add3/1, Add/2
  c/1 -> Add3/2, Add/3
  qd/1 -> Add2/2
  Add2/1 -> c/1
  Add/1 -> 1/J_CS/1
  Add1/1 -> K_torsCS/1
  1/J_CS/1 -> Integrator/1
  Add3/1 -> C1/1
  Integrator/1 -> Add2/1, Integrator1/1

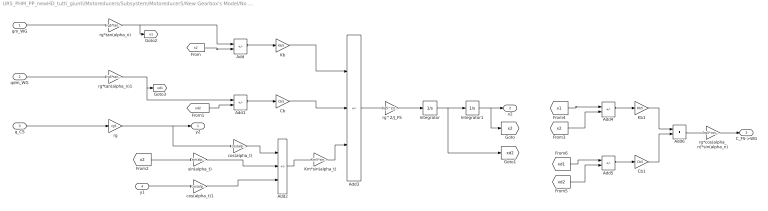
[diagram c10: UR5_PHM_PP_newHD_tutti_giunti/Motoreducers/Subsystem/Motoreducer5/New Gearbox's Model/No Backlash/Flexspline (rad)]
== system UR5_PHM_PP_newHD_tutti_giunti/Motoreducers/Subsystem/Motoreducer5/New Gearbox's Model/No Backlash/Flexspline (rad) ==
  qm_WG : Inport
  qdm_WG : Inport  Port=2
  q_CS : Inport  Port=3
  y1 : Inport  Port=4
  Add{,1,4..5} (4 alike) : Sum  Inputs=+-
  Add2 : Sum  Inputs=-+-
  Add3 : Sum  Inputs=++-
  Add6 : Sum
  Cb : Gain  Gain=Cb5
  Cb1 : Gain  Gain=Cb5
  Integrator : Integrator
  Integrator1 : Integrator  InitialCondition=x2_05
  Kb : Gain  Gain=Kb5
  Kb1 : Gain  Gain=Kb5
  Km*sin(alpha_t) : Gain  Gain=Km5*sin(alpha_t)
  cos(alpha_t) : Gain  Gain=cos(alpha_t)
  cos(alpha_t)1 : Gain  Gain=cos(alpha_t)
  rg : Gain  Gain=rg5
  rg*cos(alpha_n)*sin(alpha_n) : Gain  Gain=rg5*cos(alpha_n)*sin(alpha_n)
  rg*tan(alpha_n) : Gain  Gain=rg5*tan(alpha_n)
  rg*tan(alpha_n)1 : Gain  Gain=rg5*tan(alpha_n)
  rg^2/J_FS : Gain  Gain=rg5^2/J_FS5
  sin(alpha_t) : Gain  Gain=sin(alpha_t)
  y2 : Outport
  x2 : Outport  Port=2
  C_FS->WG : Outport  Port=3
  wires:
  Cb1/1 -> Add6/2
  Kb1/1 -> Add6/1
  sin(alpha_t)/1 -> Add2/2
  Add4/1 -> Kb1/1
  cos(alpha_t)1/1 -> Add2/3
  Add2/1 -> Km*sin(alpha_t)/1
  y1/1 -> cos(alpha_t)1/1
  Cb/1 -> Add3/2
  qdm_WG/1 -> rg*tan(alpha_n)1/1
  q_CS/1 -> rg/1
  Kb/1 -> Add3/1
  Km*sin(alpha_t)/1 -> Add3/3
  Add1/1 -> Cb/1
  rg/1 -> cos(alpha_t)/1, y2/1
  Integrator1/1 -> [x2], x2/1
  Add3/1 -> rg^2/J_FS/1
  rg^2/J_FS/1 -> Integrator/1
  cos(alpha_t)/1 -> Add2/1
  Add/1 -> Kb/1
  Integrator/1 -> [xd2], Integrator1/1
  Add5/1 -> Cb1/1
  [x2] -> sin(alpha_t)/1
  rg*tan(alpha_n)1/1 -> [xd1], Add1/1
  Add6/1 -> rg*cos(alpha_n)*sin(alpha_n)/1
  rg*cos(alpha_n)*sin(alpha_n)/1 -> C_FS->WG/1
  qm_WG/1 -> rg*tan(alpha_n)/1
  [xd2] -> Add1/2
  [x2] -> Add/2
  rg*tan(alpha_n)/1 -> [x1], Add/1
  [x2] -> Add4/2
  [x1] -> Add4/1
  [xd2] -> Add5/2
  [xd1] -> Add5/1

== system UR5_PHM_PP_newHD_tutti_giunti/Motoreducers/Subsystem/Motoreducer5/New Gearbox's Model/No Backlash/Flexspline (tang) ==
  y2 : Inport
  x2 : Inport  Port=2
  Add : Sum  Inputs=+-
  Add4 : Sum  Inputs=-+-
  Integrator : Integrator
  Integrator1 : Integrator  InitialCondition=y1_05
  Km*cos(alpha_t) : Gain  Gain=Km5*cos(alpha_t)
  Kt/rg^2 : Gain  Gain=Kt5/rg5^2
  cos(alpha_t) : Gain  Gain=cos(alpha_t)
  cos(alpha_t)2 : Gain  Gain=cos(alpha_t)
  rg^2/J_FS : Gain  Gain=rg5^2/J_FS5
  sin(alpha_t) : Gain  Gain=sin(alpha_t)
  y1 : Outport
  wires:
  Integrator/1 -> Integrator1/1
  y2/1 -> cos(alpha_t)2/1
  Integrator1/1 -> cos(alpha_t)/1, Kt/rg^2/1, y1/1
  Add4/1 -> Km*cos(alpha_t)/1
  Kt/rg^2/1 -> Add/2
  rg^2/J_FS/1 -> Integrator/1
  Add/1 -> rg^2/J_FS/1
  x2/1 -> sin(alpha_t)/1
  Km*cos(alpha_t)/1 -> Add/1
  sin(alpha_t)/1 -> Add4/2
  cos(alpha_t)2/1 -> Add4/1
  cos(alpha_t)/1 -> Add4/3

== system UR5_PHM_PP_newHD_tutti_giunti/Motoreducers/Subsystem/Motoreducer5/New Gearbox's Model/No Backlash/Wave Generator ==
  qm : Inport
  qdm : Inport  Port=2
  C_FS->WG : Inport  Port=3
  1/J_WG : Gain  Gain=1/J_WG5
  Add : Sum  Inputs=+-
  Add1 : Sum  Inputs=+-
  Add2 : Sum
  Add4 : Sum  Inputs=+-
  Integrator1 : Integrator
  Integrator2 : Integrator  InitialCondition=q_WG05
  K_torsWG : Gain  Gain=K_torsWG5
  c : Gain  Gain=c5
  Cwg->rotore : Outport
  qm_WG : Outport  Port=2
  qdm_WG : Outport  Port=3
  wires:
  K_torsWG/1 -> Add2/1
  Integrator1/1 -> qdm_WG/1, Add1/2, Integrator2/1
  Add1/1 -> c/1
  c/1 -> Add2/2
  Add4/1 -> 1/J_WG/1
  Integrator2/1 -> qm_WG/1, Add/2
  Add2/1 -> Cwg->rotore/1, Add4/1
  Add/1 -> K_torsWG/1
  1/J_WG/1 -> Integrator1/1
  C_FS->WG/1 -> Add4/2
  qdm/1 -> Add1/1
  qm/1 -> Add/1

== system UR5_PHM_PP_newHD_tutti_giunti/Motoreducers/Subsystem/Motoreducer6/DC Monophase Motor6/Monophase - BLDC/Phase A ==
  Vset : Inport
  qdm : Inport  Port=2
  Add : Sum  Inputs=-+
  Gain : Gain  Gain=Motor.kv_6
  Saturation : Saturate  UpperLimit=Motor.imax6  LowerLimit=-Motor.imax6
  Transfer Fcn : TransferFcn  Numerator=[1/Motor.R_456]  Denominator=[Motor.L_456/Motor.R_456 1]
  i : Outport  VectorParamsAs1DForOutWhenUnconnected=off
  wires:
  Gain/1 -> Add/1
  Transfer Fcn/1 -> Saturation/1
  qdm/1 -> Gain/1
  Add/1 -> Transfer Fcn/1
  Vset/1 -> Add/2
  Saturation/1 -> i/1

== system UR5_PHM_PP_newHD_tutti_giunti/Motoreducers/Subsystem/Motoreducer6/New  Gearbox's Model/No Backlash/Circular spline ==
  y1 : Inport
  y2 : Inport  Port=2
  x2 : Inport  Port=3
  q : Inport  Port=4
  qd : Inport  Port=5
  1/J_CS : Gain  Gain=1/J_CS6
  Add : Sum  Inputs=+--
  Add1 : Sum  Inputs=+-
  Add2 : Sum  Inputs=+-
  Add3 : Sum
  Add4 : Sum  Inputs=-+-
  Integrator : Integrator
  Integrator1 : Integrator  InitialCondition=q_CS06
  K_torsCS : Gain  Gain=K_torsCS6
  c : Gain  Gain=c6
  cos(alpha_t) : Gain  Gain=cos(alpha_t)
  cos(alpha_t)2 : Gain  Gain=cos(alpha_t)
  rg*Km*cos(alpha_t) : Gain  Gain=rg6*Km6*cos(alpha_t)
  sin(alpha_t) : Gain  Gain=sin(alpha_t)
  C1 : Outport
  q_CS : Outport  Port=2
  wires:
  cos(alpha_t)/1 -> Add4/3
  Add4/1 -> rg*Km*cos(alpha_t)/1
  x2/1 -> sin(alpha_t)/1
  y1/1 -> cos(alpha_t)/1
  sin(alpha_t)/1 -> Add4/2
  rg*Km*cos(alpha_t)/1 -> Add/1
  cos(alpha_t)2/1 -> Add4/1
  y2/1 -> cos(alpha_t)2/1
  Add1/1 -> K_torsCS/1
  Add/1 -> 1/J_CS/1
  Add3/1 -> C1/1
  1/J_CS/1 -> Integrator/1
  Integrator/1 -> Add2/1, Integrator1/1
  c/1 -> Add3/2, Add/3
  Add2/1 -> c/1
  Integrator1/1 -> q_CS/1, Add1/1
  K_torsCS/1 -> Add3/1, Add/2
  qd/1 -> Add2/2
  q/1 -> Add1/2

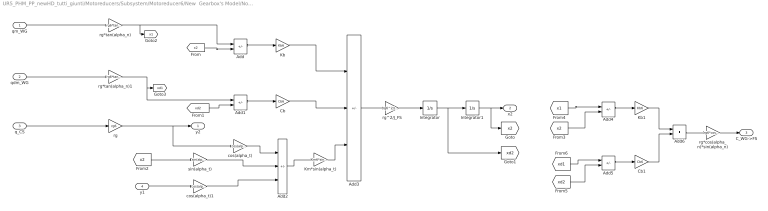
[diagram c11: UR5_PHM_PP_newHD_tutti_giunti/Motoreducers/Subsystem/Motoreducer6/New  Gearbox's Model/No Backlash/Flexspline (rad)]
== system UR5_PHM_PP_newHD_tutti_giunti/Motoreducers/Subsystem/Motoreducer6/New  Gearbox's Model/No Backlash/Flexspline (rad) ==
  qm_WG : Inport
  qdm_WG : Inport  Port=2
  q_CS : Inport  Port=3
  y1 : Inport  Port=4
  Add{,1,4..5} (4 alike) : Sum  Inputs=+-
  Add2 : Sum  Inputs=-+-
  Add3 : Sum  Inputs=++-
  Add6 : Sum
  Cb : Gain  Gain=Cb6
  Cb1 : Gain  Gain=Cb6
  Integrator : Integrator
  Integrator1 : Integrator  InitialCondition=x2_06
  Kb : Gain  Gain=Kb6
  Kb1 : Gain  Gain=Kb6
  Km*sin(alpha_t) : Gain  Gain=Km6*sin(alpha_t)
  cos(alpha_t) : Gain  Gain=cos(alpha_t)
  cos(alpha_t)1 : Gain  Gain=cos(alpha_t)
  rg : Gain  Gain=rg6
  rg*cos(alpha_n)*sin(alpha_n) : Gain  Gain=rg6*cos(alpha_n)*sin(alpha_n)
  rg*tan(alpha_n) : Gain  Gain=rg6*tan(alpha_n)
  rg*tan(alpha_n)1 : Gain  Gain=rg6*tan(alpha_n)
  rg^2/J_FS : Gain  Gain=rg6^2/J_FS6
  sin(alpha_t) : Gain  Gain=sin(alpha_t)
  y2 : Outport
  x2 : Outport  Port=2
  C_WG->FS : Outport  Port=3
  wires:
  Cb1/1 -> Add6/2
  Kb1/1 -> Add6/1
  sin(alpha_t)/1 -> Add2/2
  Add4/1 -> Kb1/1
  cos(alpha_t)1/1 -> Add2/3
  Add2/1 -> Km*sin(alpha_t)/1
  y1/1 -> cos(alpha_t)1/1
  Cb/1 -> Add3/2
  qdm_WG/1 -> rg*tan(alpha_n)1/1
  q_CS/1 -> rg/1
  Kb/1 -> Add3/1
  Km*sin(alpha_t)/1 -> Add3/3
  Add1/1 -> Cb/1
  rg/1 -> cos(alpha_t)/1, y2/1
  Integrator1/1 -> [x2], x2/1
  Add3/1 -> rg^2/J_FS/1
  rg^2/J_FS/1 -> Integrator/1
  cos(alpha_t)/1 -> Add2/1
  Add/1 -> Kb/1
  Integrator/1 -> [xd2], Integrator1/1
  Add5/1 -> Cb1/1
  [x2] -> sin(alpha_t)/1
  rg*tan(alpha_n)1/1 -> [xd1], Add1/1
  Add6/1 -> rg*cos(alpha_n)*sin(alpha_n)/1
  rg*cos(alpha_n)*sin(alpha_n)/1 -> C_WG->FS/1
  qm_WG/1 -> rg*tan(alpha_n)/1
  [xd2] -> Add1/2
  [x2] -> Add/2
  rg*tan(alpha_n)/1 -> [x1], Add/1
  [x2] -> Add4/2
  [x1] -> Add4/1
  [xd2] -> Add5/2
  [xd1] -> Add5/1

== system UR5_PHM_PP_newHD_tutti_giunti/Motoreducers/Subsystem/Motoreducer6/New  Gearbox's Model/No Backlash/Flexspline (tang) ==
  y2 : Inport
  x2 : Inport  Port=2
  Add : Sum  Inputs=+-
  Add4 : Sum  Inputs=-+-
  Integrator : Integrator
  Integrator1 : Integrator  InitialCondition=y1_06
  Km*cos(alpha_t) : Gain  Gain=Km6*cos(alpha_t)
  Kt/rg^2 : Gain  Gain=Kt6/rg6^2
  cos(alpha_t) : Gain  Gain=cos(alpha_t)
  cos(alpha_t)2 : Gain  Gain=cos(alpha_t)
  rg^2/J_FS : Gain  Gain=rg6^2/J_FS6
  sin(alpha_t) : Gain  Gain=sin(alpha_t)
  y1 : Outport
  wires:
  Integrator/1 -> Integrator1/1
  y2/1 -> cos(alpha_t)2/1
  Integrator1/1 -> cos(alpha_t)/1, Kt/rg^2/1, y1/1
  Add4/1 -> Km*cos(alpha_t)/1
  Kt/rg^2/1 -> Add/2
  rg^2/J_FS/1 -> Integrator/1
  Add/1 -> rg^2/J_FS/1
  x2/1 -> sin(alpha_t)/1
  Km*cos(alpha_t)/1 -> Add/1
  sin(alpha_t)/1 -> Add4/2
  cos(alpha_t)2/1 -> Add4/1
  cos(alpha_t)/1 -> Add4/3

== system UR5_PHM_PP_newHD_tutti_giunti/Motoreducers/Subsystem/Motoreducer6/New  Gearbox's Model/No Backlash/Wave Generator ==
  qm : Inport
  qdm : Inport  Port=2
  C_FS->WG : Inport  Port=3
  1/J_WG : Gain  Gain=1/J_WG6
  Add : Sum  Inputs=+-
  Add1 : Sum  Inputs=+-
  Add2 : Sum
  Add4 : Sum  Inputs=+-
  Integrator1 : Integrator
  Integrator2 : Integrator  InitialCondition=q_WG06
  K_torsWG : Gain  Gain=K_torsWG6
  c : Gain  Gain=c6
  Cwg->rotore : Outport
  qm_WG : Outport  Port=2
  qdm_WG : Outport  Port=3
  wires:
  Add/1 -> K_torsWG/1
  1/J_WG/1 -> Integrator1/1
  Add4/1 -> 1/J_WG/1
  Add2/1 -> Cwg->rotore/1, Add4/1
  Integrator2/1 -> qm_WG/1, Add/2
  Add1/1 -> c/1
  Integrator1/1 -> qdm_WG/1, Add1/2, Integrator2/1
  qm/1 -> Add/1
  C_FS->WG/1 -> Add4/2
  qdm/1 -> Add1/1
  K_torsWG/1 -> Add2/1
  c/1 -> Add2/2

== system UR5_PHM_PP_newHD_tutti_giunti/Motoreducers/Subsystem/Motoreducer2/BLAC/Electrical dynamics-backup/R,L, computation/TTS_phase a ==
  Tw [°C] : Inport
  Compare To Constant : simulink/Logic and Bit Operations/Compare To Constant  relop=>=  const=0.99  OutDataTypeStr=boolean
  Constant : Constant  Value=Wf_TTS_ONOFF
  Fcn : Fcn  Expr=exp(alpha_TTS*u(1))
  Fcn1 : Fcn  Expr=exp(u(1))
  Gain : Gain  Gain=Beta_TTS
  Integrator : Integrator  ExternalReset=rising
  Integrator1 : Integrator  InitialCondition=Wf_TTS_0  LimitOutput=on  UpperSaturationLimit=1  LowerSaturationLimit=0
  Multiply : Product
  Wf : Outport  VectorParamsAs1DForOutWhenUnconnected=off
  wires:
  Tw [°C]/1 -> Fcn/1
  Fcn/1 -> Gain/1
  Integrator/1 -> Integrator1/1
  Integrator1/1 -> Wf/1, Compare To Constant/1
  Compare To Constant/1 -> Integrator/2
  Fcn1/1 -> Multiply/2
  Multiply/1 -> Integrator/1
  Constant/1 -> Multiply/1
  Gain/1 -> Fcn1/1
